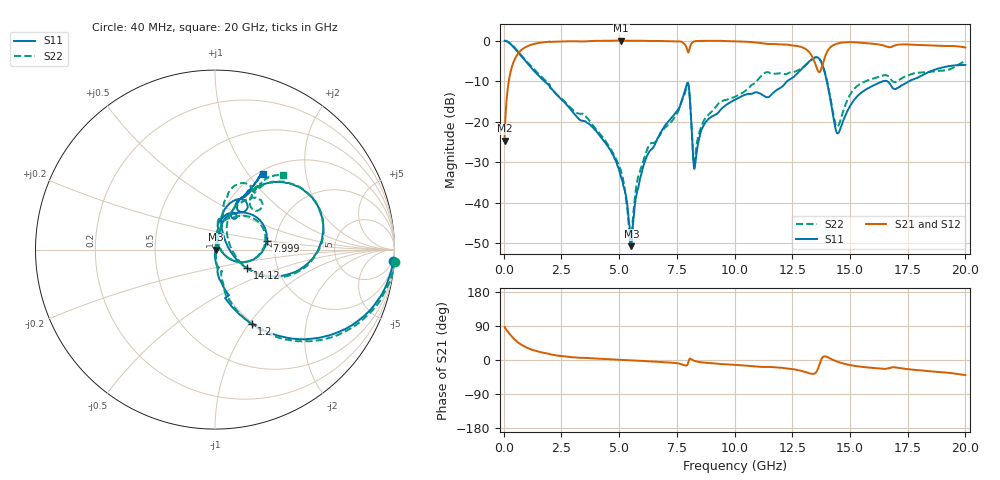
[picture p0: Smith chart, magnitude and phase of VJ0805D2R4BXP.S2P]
! VJ0805D2R4BXP
! DATE 10/29/2021  11:37
! CAPACITORS MOUNTED IN SERIES ON 25 MIL THICK MICROSTRIP SUBSTRATE
# GHz  S  MA  R  50.00
!  FREQ  S11M  S11A  S21M  S21A  S12M  S12A  S22M  S22A
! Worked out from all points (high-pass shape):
!   1601 points, 40 MHz to 20 GHz, reference 50 ohm
!   highest |S21| = -0.01 dB at 5.092 GHz (marker M1); lowest = -24.7 dB at 40 MHz (marker M2)
!   |S21| within 3 dB of the highest: 650 MHz to 13.26 GHz (12.61 GHz wide, 181 % of centre); 13.99 GHz to end of sweep
!   lowest |S11| = -50.7 dB at 5.529 GHz (marker M3), VSWR 1.01, Z = 50.3 - j0.00461 ohm
!   |S11| at or under -10 dB: 1.761 GHz to 12.28 GHz (10.52 GHz wide, 150 % of centre); 14 GHz to 16.44 GHz (2.445 GHz wide, 16.1 % of centre); 16.61 GHz to 17.57 GHz (958.4 MHz wide, 5.61 % of centre)
!   |S22| runs from -50.7 to 0.0 dB; largest |S21 - S12| = 0.0055
!   S11 on the Smith chart (normalised r, x): 40 MHz: 4, -32; 1.2 GHz: 0.98, -1.03; 7.999 GHz: 1.80, +0.20; 14.12 GHz: 1.40, -0.31; 20 GHz: 1.04, +1.18
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0.04  0.993 -3.5  0.05854 87.5  0.06038 87.1  1.004 -3.8
0.202175  0.9513 -17.0  0.292 72.9  0.2921 73.0  0.9627 -17.1
0.3893  0.8567 -30.6  0.5088 59.5  0.508 59.5  0.868 -30.8
1.200175  0.46 -63.7  0.8902 27.7  0.8906 27.6  0.4784 -62.9
3.370825  0.1034 -78.5  0.9749 5.6  0.9749 5.5  0.1257 -72.8
4.4811  0.05142 -88.1  0.9962 2.3  0.9953 2.2  0.05379 -83.7
5.092375  0.0205 -89.5  0.999 0.4  0.9981 0.3  0.02388 -80.0
5.529  0.002931 -0.9  0.997 -1.0  0.9965 -1.0  0.00344 29.4
5.865825  0.01721 65.2  0.9951 -2.0  0.9941 -2.1  0.02294 76.8
6.70165  0.06479 76.8  0.9904 -4.7  0.9899 -4.8  0.06423 78.0
7.99905  0.2925 10.0  0.7162 -5.6  0.716 -5.7  0.2853 9.8
8.285975  0.02837 45.9  0.982 -2.6  0.9815 -2.7  0.03477 52.8
8.7226  0.09686 83.7  0.9926 -7.1  0.9926 -7.2  0.1094 81.6
10.02  0.1862 75.6  0.978 -12.8  0.9764 -12.9  0.2036 77.2
12.17817  0.2932 65.5  0.8952 -21.4  0.895 -21.5  0.3868 55.1
13.35083  0.5895 35.3  0.6465 -36.5  0.6461 -36.7  0.5854 36.6
13.67517  0.5948 4.5  0.4082 -12.6  0.4084 -12.6  0.5987 4.4
14.12428  0.2072 -30.3  0.8108 4.6  0.8109 4.4  0.2175 -30.2
14.48605  0.07197 29.0  0.925 -5.1  0.9247 -5.2  0.08842 29.0
15.23455  0.1942 78.5  0.9532 -15.8  0.9527 -15.9  0.2631 64.9
16.68165  0.3049 53.3  0.8285 -21.7  0.8281 -22.1  0.3595 42.9
20  0.5003 57.9  0.8218 -39.9  0.8215 -40.2  0.5617 47.9
